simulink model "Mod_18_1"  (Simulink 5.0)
settings: Solver=ode45  StartTime=0.0  StopTime=5000  MaxStep=0.01  RelTol=1e-3
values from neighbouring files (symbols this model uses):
  Cc = 709.8    [Dados_18_1.m]
  Ci = 5923.3    [Dados_18_1.m]
  Rac = 5.215e-5    (= 5.215e-05)    [Dados_18_1.m]
  Rci = 0.1227    [Dados_18_1.m]
  Rie = 0.1226    [Dados_18_1.m]
  Ta = 80    [Dados_18_1.m]
  Tc0 = ((1+Rie/Rci)*Ta/Rac+Te/Rci)/(1/Rci+1/Rac+Rie/(Rci*Rac))    (= 79.9861841439)    [Dados_18_1.m]
  Ti0 = Te+Rie*(Ta-Tc0)/Rac    (= 47.4798458053)    [Dados_18_1.m]
libraries: simulink x1

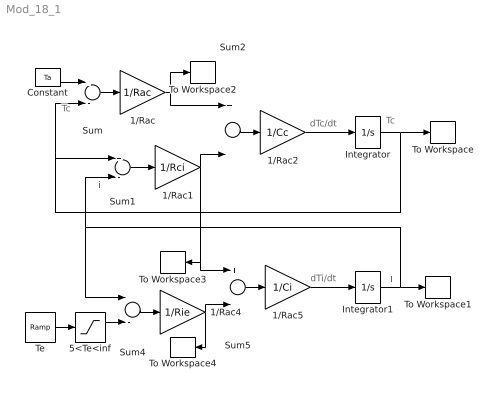
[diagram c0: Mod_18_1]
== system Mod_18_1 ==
  note: Tc
  note: Ti
  note: dTc/dt
  note: dTi/dt
  note: Tc
  note: Ti
  1/Rac : Gain  Gain=1/Rac
  1/Rac1 : Gain  Gain=1/Rci
  1/Rac2 : Gain  Gain=1/Cc
  1/Rac4 : Gain  Gain=1/Rie
  1/Rac5 : Gain  Gain=1/Ci
  5<Te<inf : Saturate  UpperLimit=inf  LowerLimit=5
  Constant : Constant  Value=Ta
  Integrator : Integrator  InitialCondition=Tc0
  Integrator1 : Integrator  InitialCondition=Ti0
  Sum{,1..2,4..5} (5 alike) : Sum  Inputs=+-
  Te : simulink/Sources/Ramp  slope=-10/3600  start=100  X0=15
  To Workspace : ToWorkspace  VariableName=Tc  SampleTime=-1  SaveFormat=Array
  To Workspace1 : ToWorkspace  VariableName=Ti  SampleTime=-1  SaveFormat=Array
  To Workspace2 : ToWorkspace  VariableName=Qac  SampleTime=-1  SaveFormat=Array
  To Workspace3 : ToWorkspace  VariableName=Qci  SampleTime=-1  SaveFormat=Array
  To Workspace4 : ToWorkspace  VariableName=Qie  SampleTime=-1  SaveFormat=Array
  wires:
  Constant/1 -> Sum/1
  Sum/1 -> 1/Rac/1
  Sum1/1 -> 1/Rac1/1
  1/Rac/1 -> Sum2/1, To Workspace2/1
  1/Rac1/1 -> Sum2/2, Sum5/1, To Workspace3/1
  Sum2/1 -> 1/Rac2/1
  1/Rac2/1 -> Integrator/1
  Te/1 -> 5<Te<inf/1
  Sum4/1 -> 1/Rac4/1
  1/Rac4/1 -> Sum5/2, To Workspace4/1
  Sum5/1 -> 1/Rac5/1
  1/Rac5/1 -> Integrator1/1
  Integrator/1 -> To Workspace/1, Sum1/1, Sum/2
  Integrator1/1 -> Sum4/1, Sum1/2, To Workspace1/1
  5<Te<inf/1 -> Sum4/2
